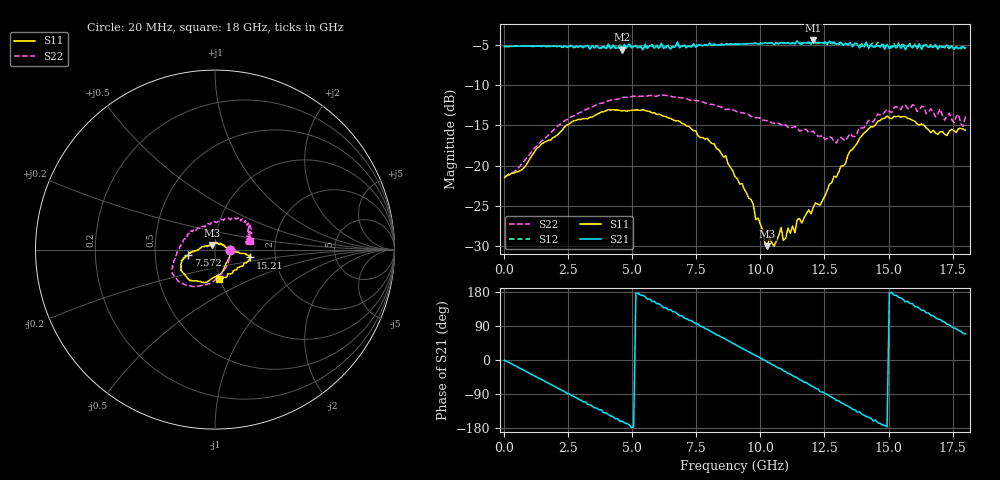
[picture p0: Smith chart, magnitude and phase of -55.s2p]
!Agilent Technologies,N5230A,US43500223,A.07.50.48
!Agilent N5230A: A.07.50.48
!Date: Tuesday, January 12, 2016 18:21:40
!Correction: S11(Full 2 Port(1,2))
!S21(Full 2 Port(1,2))
!S12(Full 2 Port(1,2))
!S22(Full 2 Port(1,2))
!S2P File: Measurements: S11, S21, S12, S22:
# Hz S  dB  R 50
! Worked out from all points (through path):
!   201 points, 20 MHz to 18 GHz, reference 50 ohm
!   highest |S21| = -4.43 dB at 12.07 GHz (marker M1); lowest = -5.6 dB at 4.605 GHz (marker M2)
!   group delay of S21, straight-line fit = 100 ps
!   lowest |S11| = -30.0 dB at 10.27 GHz (marker M3), VSWR 1.06, Z = 48.2 + j2.55 ohm
!   |S11| at or under -10 dB: start of sweep to end of sweep
!   |S22| runs from -21.4 to -11.2 dB; largest |S21 - S12| = 0.05
!   S11 on the Smith chart (normalised r, x): 20 MHz: 1.18, -0.01; 7.572 GHz: 0.74, -0.05; 15.21 GHz: 1.49, -0.13; 18 GHz: 0.99, -0.34
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2e7  -21.51 -2.9  -5.19 -0.6  -5.18 -0.8  -21.37 -1.9
9.19e8  -19.64 -56.8  -5.11 -32.4  -5.12 -32.6  -18.89 -55.7
1.818e9  -16.82 -84.0  -5.16 -64.7  -5.13 -65.5  -15.93 -86.3
3.0766e9  -14.17 -111.1  -5.35 -110.2  -5.27 -110.0  -13.25 -112.3
4.0655e9  -13.04 -128.9  -4.86 -143.8  -5.12 -143.0  -11.94 -127.9
4.6049e9  -13.21 -137.0  -5.58 -161.2  -5.41 -163.7  -11.56 -134.2
5.5039e9  -13.15 -149.2  -4.89 167.2  -5.27 167.7  -11.34 -144.9
6.0433e9  -13.59 -156.2  -5.38 148.0  -5.49 145.8  -11.25 -149.9
6.7625e9  -14.41 -163.0  -4.61 121.8  -4.91 121.7  -11.54 -154.8
7.5716e9  -16.33 -167.8  -4.97 94.7  -5.04 93.8  -11.93 -159.1
9.01e9  -21.39 175.6  -4.86 41.6  -4.86 40.6  -13.17 -171.5
9.6393e9  -24.26 161.0  -4.82 17.9  -4.82 17.4  -13.87 -179.8
1.02686e10  -30.05 123.1  -4.78 -5.4  -4.80 -5.6  -14.41 171.3
1.13474e10  -28.38 57.0  -4.89 -44.7  -4.79 -45.6  -15.15 151.5
1.14373e10  -26.73 46.7  -4.47 -46.8  -4.76 -48.8  -15.29 148.2
1.20666e10  -25.19 24.3  -4.43 -70.9  -4.71 -72.3  -15.72 137.1
1.3505e10  -18.18 -7.2  -4.69 -125.2  -4.73 -125.5  -16.01 92.6
1.41343e10  -15.73 -7.6  -4.62 -149.0  -4.95 -148.6  -14.87 72.3
1.50333e10  -14.08 -10.1  -5.44 176.9  -5.20 175.8  -13.25 47.8
1.52131e10  -13.87 -12.4  -5.10 171.0  -4.76 170.7  -12.80 48.5
1.66515e10  -15.91 -39.1  -5.14 117.7  -4.95 116.2  -12.95 29.0
1.8e10  -15.59 -82.2  -5.36 68.6  -5.46 65.5  -13.89 13.3
